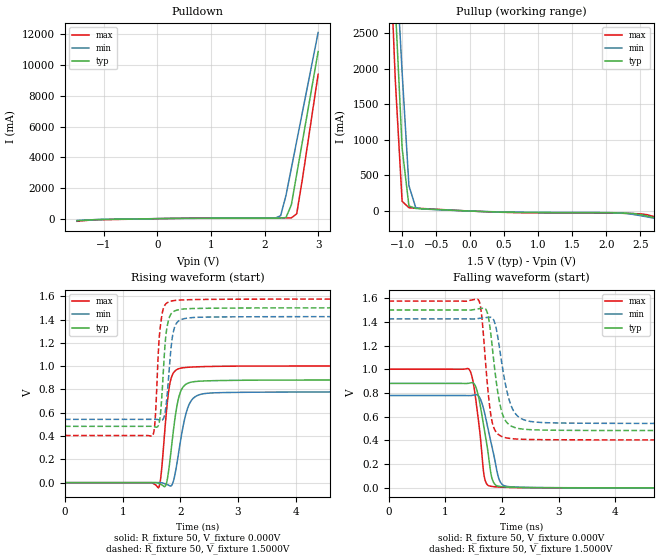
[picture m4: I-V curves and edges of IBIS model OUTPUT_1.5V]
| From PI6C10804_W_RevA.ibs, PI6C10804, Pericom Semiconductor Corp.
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|   Model OUTPUT
[Model]   OUTPUT_1.5V
Model_type Output
Cref=50p
Vmeas=425mV
| variable   typ   min   max
C_comp   1.150pF   1.149pF   1.151pF
[Voltage Range]   1.5000V   1.4250V   1.5750V
[POWER Clamp Reference]   1.5000V   1.4250V   1.5750V
[GND Clamp Reference]   0.0000V   0.0000V   0.0000V
[Pullup Reference]   1.5000V   1.4250V   1.5750V
[Pulldown Reference]   0.0000V   0.0000V   0.0000V
[Temperature Range]   25   85   -40
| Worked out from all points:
|   slope of the pulldown table from 0 to 0.225 V, typ, clamps not added: 20.6 ohm
|   slope of the pullup table from 0 to 0.225 V, typ, clamps not added: 28.1 ohm
|   falling waveform, R_fixture 50, V_fixture 0.000V: 20-80 % time 175ps typ, 208ps min, 140ps max; typ from 0.881 V to 0 V
|   rising waveform, R_fixture 50, V_fixture 0.000V: 20-80 % time 144ps typ, 178ps min, 111ps max; typ from 0 V to 0.881 V
|   falling waveform, R_fixture 50, V_fixture 1.5000V: 20-80 % time 170ps typ, 208ps min, 132ps max; typ from 1.5 V to 0.483 V
|   rising waveform, R_fixture 50, V_fixture 1.5000V: 20-80 % time 86.5ps typ, 96.8ps min, 78.5ps max; typ from 0.483 V to 1.5 V
[Pulldown]
| Voltage   I(typ)   I(min)   I(max)
-1.5V     -137.6mA   -120.7mA   -172.9mA
-1.1V     -59.46mA   -55.51mA   -71.52mA
200mV     9.891mA    7.906mA    13.05mA
2.1V      32.33mA    28.32mA    39.31mA
2.2V      34.02mA    37.09mA    40.29mA
2.3V      36.94mA    191.8mA    42.13mA
2.4V      70.56mA    1.513A     44.67mA
2.5V      895mA      3.281A     50.1mA
2.6V      2.893A     5.049A     314.4mA
2.7V      4.89A      6.817A     2.432A
3V        10.88A     12.12A     9.407A
[Pullup]
| Voltage   I(typ)   I(min)   I(max)
-1.5V     10.88A     10.79A     11.14A
-1.2V     4.882A     5.488A     4.16A
-1.1V     2.884A     3.719A     1.835A
-1V       885.7mA    1.95A      137mA
-900mV    71.66mA    356.4mA    46.24mA
-800mV    36.69mA    48.28mA    40.46mA
-700mV    31.31mA    29.16mA    35.34mA
600mV     -17.29mA   -14.92mA   -20.6mA
2.1V      -25.5mA    -23.43mA   -29.57mA
2.5V      -49.25mA   -64.36mA   -39.3mA
2.7V      -90.84mA   -99.22mA   -76.91mA
3V        -160.5mA   -154.1mA   -175mA
[Falling Waveform]
R_fixture = 50
V_fixture = 0.000V
V_fixture_min = 0.000V
V_fixture_max = 0.000V
|   Time   V(typ)   V(min)   V(max)
0s        881mV      778.7mV    1.001V
1.42ns    882.6mV    777.9mV    1.002V
1.492ns   885.4mV    781.1mV    894.7mV
1.572ns   801.5mV    781.6mV    624.4mV
1.684ns   510.6mV    654.1mV    110.9mV
1.79ns    174.7mV    423.3mV    15.02mV
1.85ns    49.17mV    294.1mV    10.5mV
1.95ns    13.11mV    73.9mV     6.581mV
2.1ns     6.627mV    11.66mV    3.794mV
9.8ns     0V         939.9nV    0V
[Rising Waveform]
R_fixture = 50
V_fixture = 0.000V
V_fixture_min = 0.000V
V_fixture_max = 0.000V
|   Time   V(typ)   V(min)   V(max)
0s        0V         0V         0V
1.621ns   -5.845mV   631.1uV    -44.77mV
1.67ns    -17.04mV   -30.74uV   80mV
1.747ns   -24.49mV   -12.09mV   536.7mV
1.818ns   177.8mV    -26.75mV   844.7mV
1.89ns    483.1mV    29.24mV    947.7mV
2.01ns    786.6mV    375.5mV    982.7mV
2.18ns    861.5mV    695.3mV    991.5mV
2.46ns    873.5mV    766.5mV    996.5mV
10ns      881mV      778.7mV    1.001V
[Falling Waveform]
R_fixture = 50
V_fixture = 1.5000V
V_fixture_min = 1.4250V
V_fixture_max = 1.5750V
|   Time   V(typ)   V(min)   V(max)
0s        1.5V       1.425V     1.575V
1.58ns    1.51V      1.428V     1.59V
1.64ns    1.513V     1.432V     1.471V
1.73ns    1.495V     1.437V     953.8mV
1.82ns    1.233V     1.436V     575.9mV
1.93ns    801.6mV    1.267V     453.9mV
2.04ns    587.4mV    932.3mV    426.2mV
2.22ns    509.8mV    638.7mV    413.2mV
2.6ns     488.9mV    554.4mV    407.2mV
9.8ns     483.3mV    543.2mV    404.7mV
[Rising Waveform]
R_fixture = 50
V_fixture = 1.5000V
V_fixture_min = 1.4250V
V_fixture_max = 1.5750V
|   Time   V(typ)   V(min)   V(max)
0s        483.3mV    543.2mV    404.7mV
1.52ns    482.8mV    543.6mV    402.7mV
1.565ns   478.1mV    543.5mV    543.7mV
1.625ns   497mV      539.8mV    1.169V
1.66ns    608.4mV    535.6mV    1.362V
1.745ns   1.236V     630mV      1.531V
1.83ns    1.44V      1.102V     1.556V
1.92ns    1.477V     1.357V     1.564V
2.14ns    1.493V     1.413V     1.57V
8ns       1.5V       1.425V     1.575V
[Ramp]
| variable   typ   min   max
dV/dt_r   0.52819V/143.96p   0.46664V/178.15p   0.59973V/111.09p
dV/dt_f   0.66324V/169.71p   0.52838V/207.94p   0.70206V/132.35p
R_load = 50
